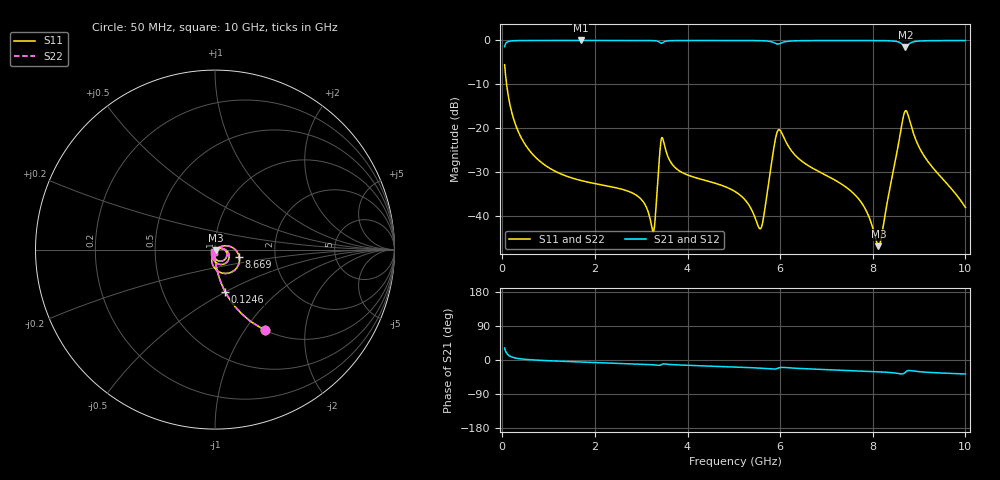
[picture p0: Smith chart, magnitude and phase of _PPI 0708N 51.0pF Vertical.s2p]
! S-Parameter data specifications (vertical orientation):
! Substrate: 40-mil Rogers 3003C, Substrate thickness, H=1.016mm, Dielectric constant, Er=3, Conductor thickness, T_mtl=0.043mm, Loss Tangent, Tand=0.003
! PCB Mounting Pad Footprint: Pad width, PadW=2.54mm , Pad length, PadL=0.51mm , Pad gap, PadG (edge-to-edge)=0.71mm , Reference planes=1.73mm apart
! Created Tue Jan 16 08:53:41 2018
# GHz S MA R 50
! 2 Port Network Data from SP1.SP block
! freq  magS11  angS11  magS21  angS21  magS12  angS12  magS22  angS22
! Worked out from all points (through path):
!   801 points, 50 MHz to 10 GHz, reference 50 ohm
!   highest |S21| = -0.01 dB at 1.692 GHz (marker M1); lowest = -1.5 dB at 8.707 GHz (marker M2)
!   group delay of S21, straight-line fit = 11.2 ps
!   lowest |S11| = -46.9 dB at 8.122 GHz (marker M3), VSWR 1.01, Z = 50.3 - j0.318 ohm
!   |S11| at or under -10 dB: 93.56 MHz to end of sweep
!   |S22| runs from -46.9 to -5.5 dB; largest |S21 - S12| = 0
!   S11 on the Smith chart (normalised r, x): 50 MHz: 1.00, -1.24; 124.6 MHz: 1.00, -0.50; 8.669 GHz: 1.31, -0.11; 10 GHz: 0.99, -0.02
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0.05  0.5282 -58.3  0.849 31.7  0.849 31.7  0.5282 -58.3
0.124625  0.2426 -76.4  0.97 13.5  0.97 13.5  0.2426 -76.4
0.3111875  0.1008 -85.3  0.9947 4.6  0.9947 4.6  0.1008 -85.3
0.6096875  0.05368 -89.0  0.9983 0.7  0.9983 0.7  0.05368 -89.0
1.69175  0.02533 -94.2  0.9991 -5.2  0.9991 -5.2  0.02533 -94.2
1.716625  0.02514 -94.3  0.9991 -5.3  0.9991 -5.3  0.02514 -94.3
2.88575  0.01731 -97.1  0.9987 -10.4  0.9987 -10.4  0.01731 -97.1
3.246437  0.006781 -55.5  0.9949 -12.5  0.9949 -12.5  0.006781 -55.5
3.370812  0.03164 13.3  0.9717 -14.1  0.9717 -14.1  0.03164 13.3
3.470312  0.07433 -59.5  0.9496 -10.4  0.9496 -10.4  0.07433 -59.5
3.806125  0.03301 -98.8  0.9969 -13.0  0.9969 -13.0  0.03301 -98.8
5.025  0.01894 -103.3  0.9979 -18.5  0.9979 -18.5  0.01894 -103.3
5.584688  0.007218 -38.0  0.9928 -21.6  0.9928 -21.6  0.007218 -38.0
5.982687  0.09609 -51.3  0.9161 -20.4  0.9161 -20.4  0.09609 -51.3
6.691625  0.03515 -108.0  0.9955 -23.8  0.9955 -23.8  0.03515 -108.0
7.66175  0.01635 -109.5  0.997 -28.5  0.997 -28.5  0.01635 -109.5
8.121937  0.00451 -44.5  0.9953 -31.0  0.9953 -31.0  0.00451 -44.5
8.345812  0.01775 26.6  0.9905 -32.7  0.9905 -32.7  0.01775 26.6
8.669187  0.1419 -17.4  0.8638 -35.5  0.8638 -35.5  0.1419 -17.4
8.7065  0.1584 -39.5  0.8425 -31.9  0.8425 -31.9  0.1584 -39.5
9.1045  0.04854 -111.4  0.9897 -31.8  0.9897 -31.8  0.04854 -111.4
10  0.01245 -115.1  0.997 -37.0  0.997 -37.0  0.01245 -115.1
